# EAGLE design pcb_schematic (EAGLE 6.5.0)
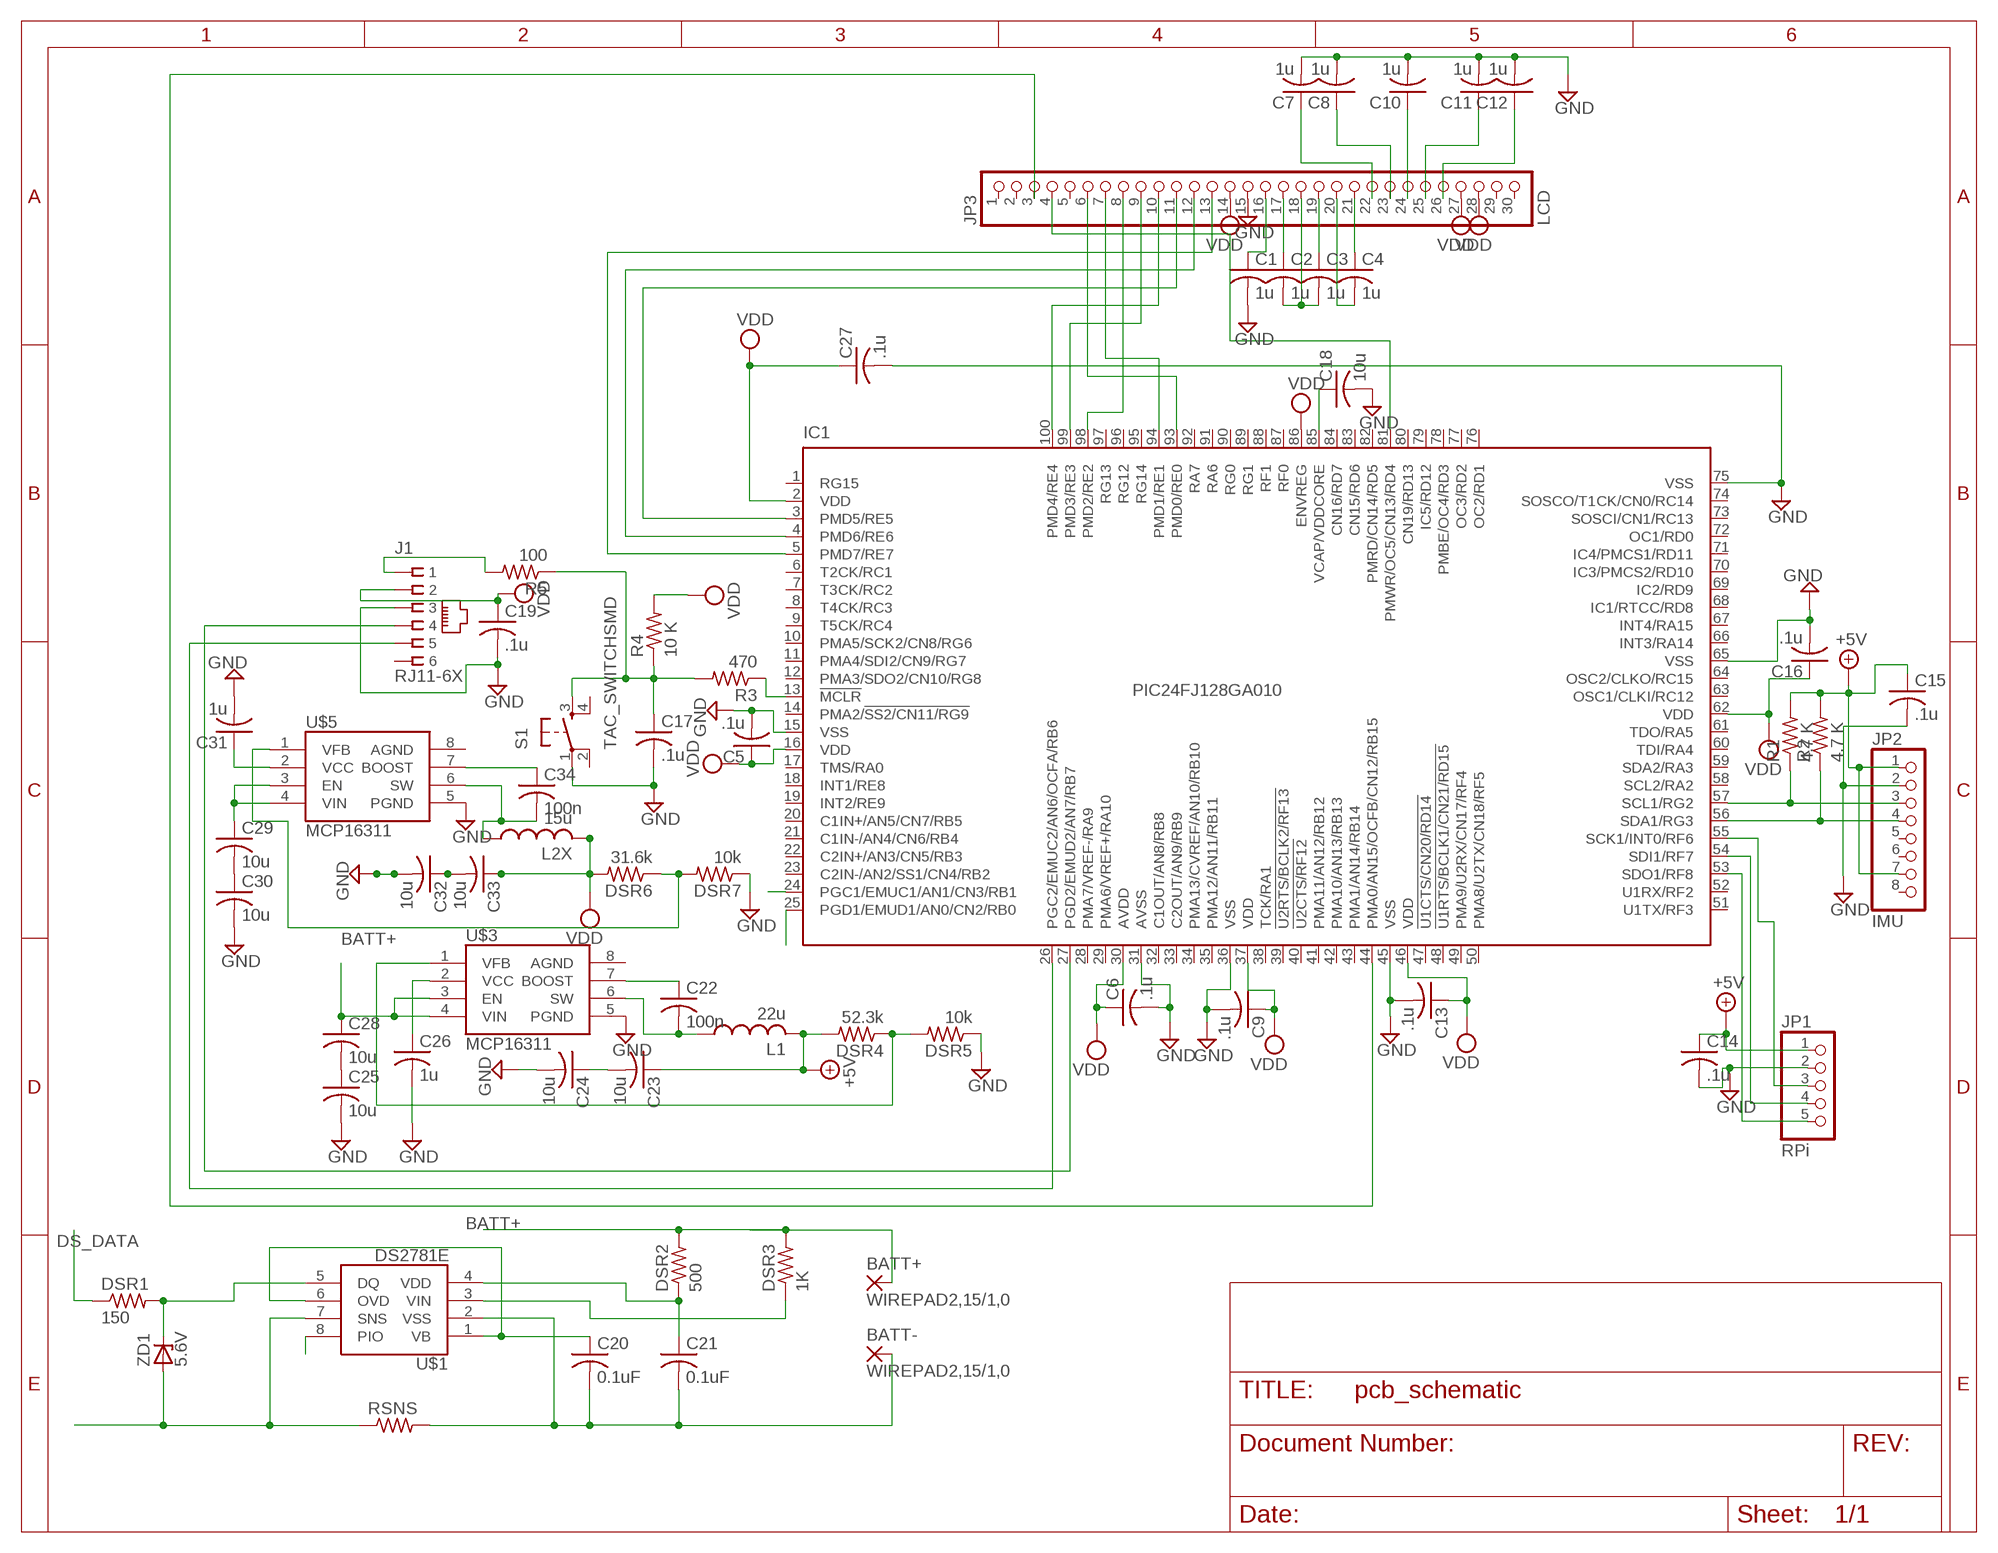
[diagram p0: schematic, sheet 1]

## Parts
BATT+  WIREPAD2,15/1,0  [2,15/1,0]
BATT-  WIREPAD2,15/1,0  [2,15/1,0]
C1  1u  C-USC1206K  [C1206K]
C2  1u  C-USC1206K  [C1206K]
C3  1u  C-USC1206K  [C1206K]
C4  1u  C-USC1206K  [C1206K]
C5  .1u  C-USC1206K  [C1206K]
C6  .1u  C-USC1206K  [C1206K]
C7  1u  C-USC1206K  [C1206K]
C8  1u  C-USC1206K  [C1206K]
C9  .1u  C-USC1206K  [C1206K]
C10  1u  C-USC1206K  [C1206K]
C11  1u  C-USC1206K  [C1206K]
C12  1u  C-USC1206K  [C1206K]
C13  .1u  C-USC1206K  [C1206K]
C14  .1u  C-USC1206K  [C1206K]
C15  .1u  C-USC1206K  [C1206K]
C16  .1u  C-USC1206K  [C1206K]
C17  .1u  C-USC1206K  [C1206K]
C18  10u  C-USC1206K  [C1206K]
C19  .1u  C-USC1206K  [C1206K]
C20  0.1uF  C-US025-024X044  [C025-024X044]
C21  0.1uF  C-US025-024X044  [C025-024X044]
C22  100n  C-US025-024X044  [C025-024X044]
C23  10u  C-US025-024X044  [C025-024X044]
C24  10u  C-US025-024X044  [C025-024X044]
C25  10u  C-US025-024X044  [C025-024X044]
C26  1u  C-US025-024X044  [C025-024X044]
C27  .1u  C-USC1206K  [C1206K]
C28  10u  C-US025-024X044  [C025-024X044]
C29  10u  C-US025-024X044  [C025-024X044]
C30  10u  C-US025-024X044  [C025-024X044]
C31  1u  C-US025-024X044  [C025-024X044]
C32  10u  C-US025-024X044  [C025-024X044]
C33  10u  C-US025-024X044  [C025-024X044]
C34  100n  C-US025-024X044  [C025-024X044]
DSR1  150  R-US_M2012  [M2012]
DSR2  500  R-US_M2012  [M2012]
DSR3  1K  R-US_M2012  [M2012]
DSR4  52.3k  R-US_M2012  [M2012]
DSR5  10k  R-US_M2012  [M2012]
DSR6  31.6k  R-US_M2012  [M2012]
DSR7  10k  R-US_M2012  [M2012]
IC1  PIC24FJ128GA010  [TQFP100-14X14]
J1  RJ11-6X  [RJ11-NO_SHIELD]
JP1  RPi  PINHD-1X5  [1X05]
JP2  IMU  PINHD-1X8  [1X08]
JP3  LCD  PINHD-1X30  [1X30]
L1  22u  L-US0204/5  [0204/5]
L2X  15u  L-US0204/5  [0204/5]
R1  4.7 K  R-US_M2012  [M2012]
R2  4.7 K  R-US_M2012  [M2012]
R3  470  R-US_M2012  [M2012]
R4  10 K  R-US_M2012  [M2012]
R5  100  R-US_M2012  [M2012]
RSNS  R-US_M2012  [M2012]
S1  TAC_SWITCHSMD  [TACTILE-SWITCH-SMD]
U$1  DS2781E  [TSSOP8]
U$3  MCP16311  [MSOP8]
U$5  MCP16311  [MSOP8]
ZD1  5.6V  ZENER-DIODESOD80C  [SOD80C]

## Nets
+5V: C14.1 C15.1 C23.1 DSR4.2 JP1.1 JP2.1 JP2.7 L1.2 R1.2 R2.2
BATT+: BATT+.1(P) C28.1 C29.1 DSR2.2 DSR3.2 U$3.3(EN) U$3.4(VIN) U$5.3(EN) U$5.4(VIN)
DS_DATA: DSR1.1 IC1.25(PGD1/EMUD1/AN0/CN2/RB0)
DS_PACK-: RSNS.1 U$1.7(SNS) ZD1.A
GND: C1.2 C5.2 C6.2 C7.2 C8.2 C9.2 C10.2 C11.2 C12.2 C13.2 C14.2 C15.2 C16.2 C17.2 C18.2 C19.2 C24.2 C25.2 C26.2 C27.2 C30.2 C31.2 C32.2 DSR5.1 DSR7.1 IC1.15(VSS) IC1.31(AVSS) IC1.36(VSS) IC1.45(VSS) IC1.65(VSS) IC1.75(VSS) J1.3 JP1.2 JP2.2 JP3.15 S1.1 U$3.5(PGND) U$5.5(PGND)
N$1: IC1.57(SCL1/RG2) JP2.3 R1.1
N$2: IC1.56(SDA1/RG3) JP2.4 R2.1
N$3: IC1.44(PMA0/AN15/OCFB/CN12/RB15) JP3.3
N$4: IC1.55(SCK1/INT0/RF6) JP1.3
N$5: IC1.54(SDI1/RF7) JP1.4
N$6: IC1.53(SDO1/RF8) JP1.5
N$7: C18.1 IC1.85(VCAP/VDDCORE)
N$8: IC1.5(PMD7/RE7) JP3.13
N$9: IC1.4(PMD6/RE6) JP3.12
N$10: IC1.3(PMD5/RE5) JP3.11
N$11: IC1.100(PMD4/RE4) JP3.10
N$12: IC1.99(PMD3/RE3) JP3.9
N$13: IC1.98(PMD2/RE2) JP3.8
N$14: IC1.94(PMD1/RE1) JP3.7
N$15: IC1.93(PMD0/RE0) JP3.6
N$16: C7.1 JP3.22
N$17: C3.1 JP3.19
N$18: IC1.81(PMWR/OC5/CN13/RD4) JP3.4
N$19: C2.1 JP3.17
N$20: C2.2 C3.2 JP3.18
N$21: C1.1 JP3.16
N$22: C4.2 JP3.20
N$23: C4.1 JP3.21
N$24: C8.1 JP3.23
N$25: C10.1 JP3.24
N$26: C11.1 JP3.25
N$27: C12.1 JP3.26
N$29: J1.1 R5.2
N$30: C25.1 C28.2
N$31: DSR1.2 U$1.5(DQ) ZD1.C
N$32: IC1.26(PGC2/EMUC2/AN6/OCFA/RB6) J1.5
N$33: IC1.27(PGD2/EMUD2/AN7/RB7) J1.4
N$34: C17.1 R3.2 R4.1 R5.1 S1.3
N$35: BATT-.1(P) C20.2 C21.2 RSNS.2 U$1.2(VSS)
N$36: C21.1 DSR2.1 U$1.4(VDD)
N$37: C20.1 U$1.1(VB) U$1.6(OVD)
N$38: C22.2 L1.1 U$3.6(SW)
N$39: DSR3.1 U$1.3(VIN)
N$40: C22.1 U$3.7(BOOST)
N$41: DSR4.1 DSR5.2 U$3.1(VFB)
N$42: C23.2 C24.1
N$43: C26.1 U$3.2(VCC)
N$44: C29.2 C30.1
N$45: C32.1 C33.2
N$46: DSR6.1 DSR7.2 U$5.1(VFB)
N$47: C34.2 L2X.1 U$5.6(SW)
N$48: C34.1 U$5.7(BOOST)
N$49: C31.1 U$5.2(VCC)
N$50: IC1.13(!MCLR) R3.1
PIO: IC1.24(PGC1/EMUC1/AN1/CN3/RB1) U$1.8(PIO)
VDD: C5.1 C6.1 C9.1 C13.1 C16.1 C19.1 C27.1 C33.1 DSR6.2 IC1.2(VDD) IC1.16(VDD) IC1.30(AVDD) IC1.37(VDD) IC1.46(VDD) IC1.62(VDD) IC1.86(ENVREG) J1.2 JP3.14 JP3.27 JP3.28 L2X.2 R4.2
Unconnected: IC1.1(RG15) IC1.6(T2CK/RC1) IC1.7(T3CK/RC2) IC1.8(T4CK/RC3) IC1.9(T5CK/RC4) IC1.10(PMA5/SCK2/CN8/RG6) IC1.11(PMA4/SDI2/CN9/RG7) IC1.12(PMA3/SDO2/CN10/RG8) IC1.14(PMA2/!SS2/CN11/RG9) IC1.17(TMS/RA0) IC1.18(INT1/RE8) IC1.19(INT2/RE9) IC1.20(C1IN+/AN5/CN7/RB5) IC1.21(C1IN-/AN4/CN6/RB4) IC1.22(C2IN+/AN3/CN5/RB3) IC1.23(C2IN-/AN2/SS1/CN4/RB2) IC1.28(PMA7/VREF-/RA9) IC1.29(PMA6/VREF+/RA10) IC1.32(C1OUT/AN8/RB8) IC1.33(C2OUT/AN9/RB9) IC1.34(PMA13/CVREF/AN10/RB10) IC1.35(PMA12/AN11/RB11) IC1.38(TCK/RA1) IC1.39(!U2RTS/BCLK2/RF13) IC1.40(!U2CTS/RF12) IC1.41(PMA11/AN12/RB12) IC1.42(PMA10/AN13/RB13) IC1.43(PMA1/AN14/RB14) IC1.47(!U1CTS/CN20/RD14) IC1.48(!U1RTS/BCLK1/CN21/RD15) IC1.49(PMA9/U2RX/CN17/RF4) IC1.50(PMA8/U2TX/CN18/RF5) IC1.51(U1TX/RF3) IC1.52(U1RX/RF2) IC1.58(SCL2/RA2) IC1.59(SDA2/RA3) IC1.60(TDI/RA4) IC1.61(TDO/RA5) IC1.63(OSC1/CLKI/RC12) IC1.64(OSC2/CLKO/RC15) IC1.66(INT3/RA14) IC1.67(INT4/RA15) IC1.68(IC1/RTCC/RD8) IC1.69(IC2/RD9) IC1.70(IC3/PMCS2/RD10) IC1.71(IC4/PMCS1/RD11) IC1.72(OC1/RD0) IC1.73(SOSCI/CN1/RC13) IC1.74(SOSCO/T1CK/CN0/RC14) IC1.76(OC2/RD1) IC1.77(OC3/RD2) IC1.78(PMBE/OC4/RD3) IC1.79(IC5/RD12) IC1.80(CN19/RD13) IC1.82(PMRD/CN14/RD5) IC1.83(CN15/RD6) IC1.84(CN16/RD7) IC1.87(RF0) IC1.88(RF1) IC1.89(RG1) IC1.90(RG0) IC1.91(RA6) IC1.92(RA7) IC1.95(RG14) IC1.96(RG12) IC1.97(RG13) J1.6 JP2.5 JP2.6 JP2.8 JP3.1 JP3.2 JP3.5 JP3.29 JP3.30 S1.2 S1.4 U$3.8(AGND) U$5.8(AGND)

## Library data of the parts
BATT+ BATT- = wirepad:WIREPAD: Wire PAD connect wire on PCB
C1-C34 = rcl:C-US: CAPACITOR, American symbol
DSR1-DSR7 R1-R5 RSNS = rcl:R-US_: RESISTOR, American symbol
IC1 = microchip:PIC24FJ*GA010: 64/80/100-Pin General Purpose, 16-Bit Flash Microcontrollers Source: http://ww1.microchip.com/downloads/en/DeviceDoc/39747d.pdf; MPN: PIC24FJ128GA010-I/PT; OC_FARNELL: 1146522; OC_NEWARK: 56K7341
J1 = con-tycoelectronics:RJ11: CORCOM Modular RJ Jacks No Shield Source: www.tycoelectronics.com .. ENG_DS_1654001_1099_RJ_L_0507.pdf; MPN: RJ11-6X; OC_FARNELL: unknown; OC_NEWARK: 16R6089
JP1 = pinhead:PINHD-1X5: PIN HEADER
JP2 = pinhead:PINHD-1X8: PIN HEADER
JP3 = pinhead:PINHD-1X30: PIN HEADER
L1 L2X = rcl:L-US: INDUCTOR, American symbol
S1 = SparkFun-Retired:TAC_SWITCH: Momentary Switch Button commonly used for reset or general input. Spark Fun Electronics SKU : COM-00097 SMT- SWCH-08247; PROD_ID: SWCH-08247
U$1 = fuelgauge:DS2781E
U$3 U$5 = fuelgauge:MCP16311
ZD1 = diode:ZENER-DIODE: Z-Diode

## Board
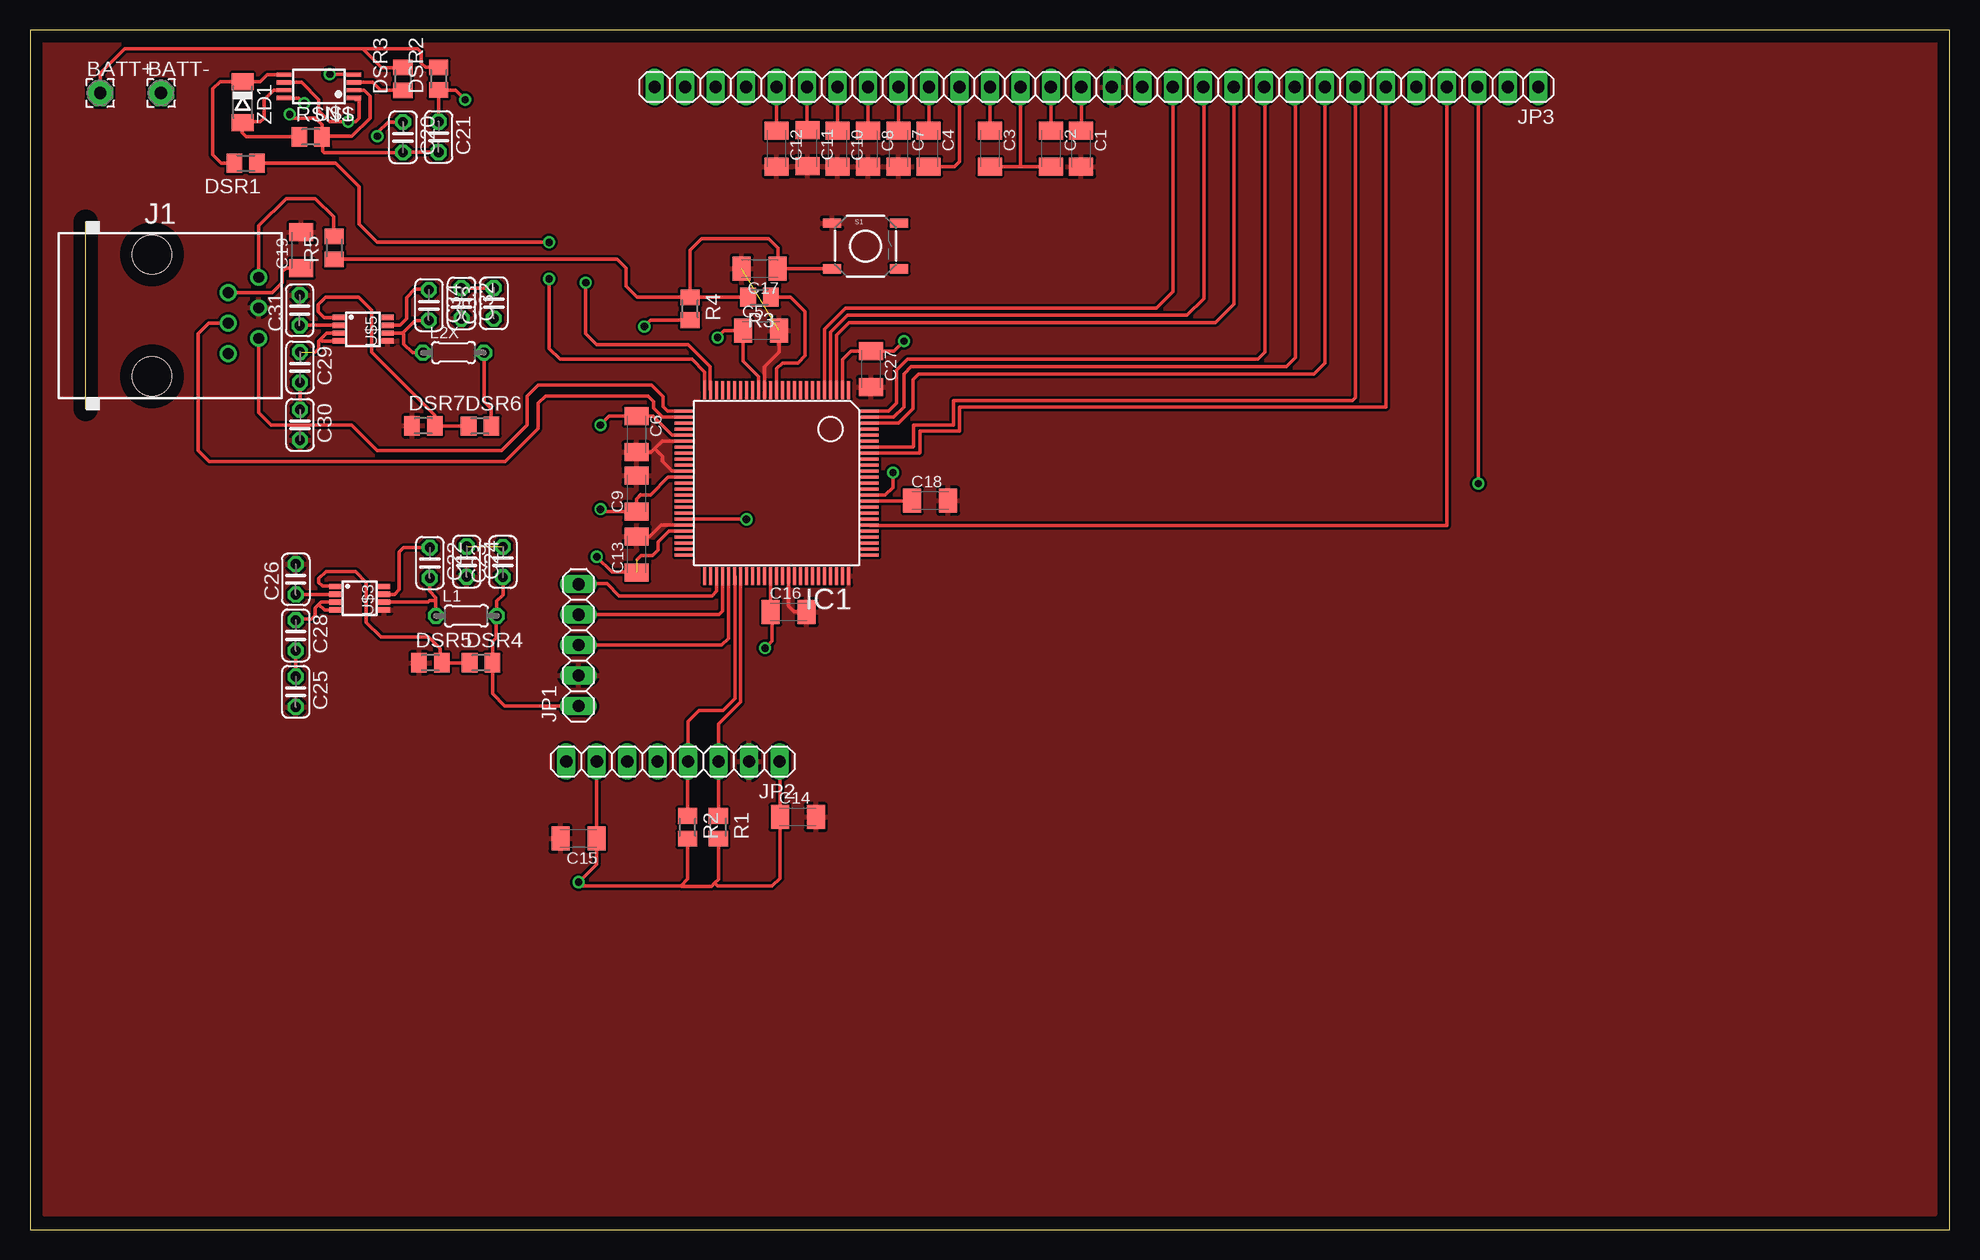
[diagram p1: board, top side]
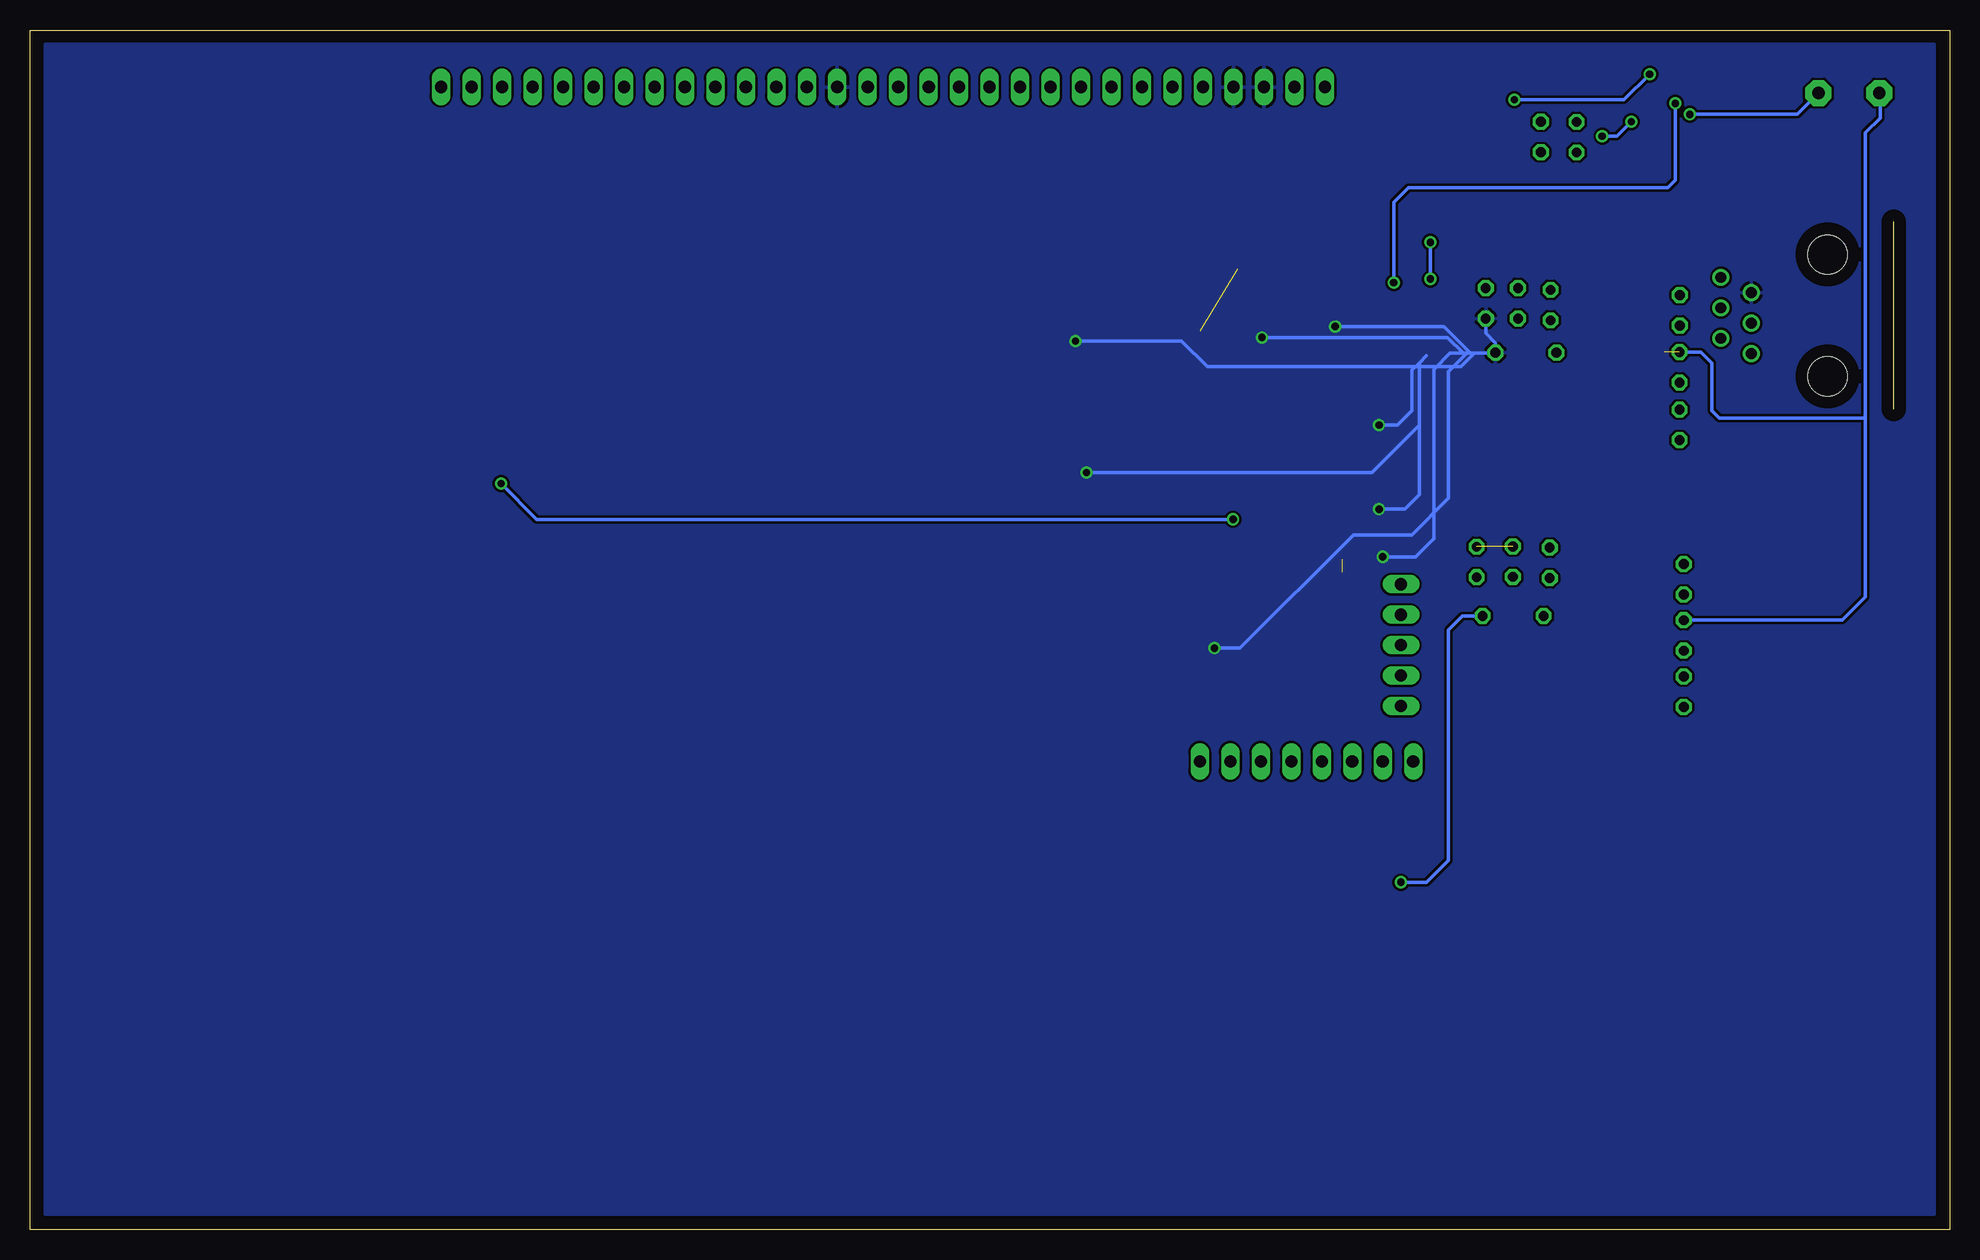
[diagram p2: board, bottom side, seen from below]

Size 160 x 100 mm. Coordinates in mm from the lower left corner, seen from the top.
Outline: 0,0 160,0 160,100 0,100 0,0
Copper layers (1*16): Top 0.035mm / dielectric 1.5mm / Bottom 0.035mm
Design rules "default": minimum track width 10mil, minimum drill 24mil, track to track 8mil, track to pad 8mil, pad to pad 8mil, via to via 8mil, smd to smd 8mil, copper to edge 40mil, drill to drill 8mil, minimum pad ring 10mil, minimum via ring 8mil, stop-mask expansion 4mil, vias tented up to drill 0mil, thermal gap 10mil

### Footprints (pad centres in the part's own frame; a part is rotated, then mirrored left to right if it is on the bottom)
2,15/1,0 = drill 1.016 pad 2.159 octagon: 1 0,0
C1206K = smd 1.5 x 2: 1 -1.5,0; 2 1.5,0
C025-024X044 = drill 0.813 octagon: 1 -1.27,0; 2 1.27,0
M2012 = smd 1.3 x 1.6: 1 -0.95,0; 2 0.95,0
TQFP100-14X14 = smd 0.27 x 1.5: 1 -6,-7.75; 2 -5.5,-7.75; 3 -5,-7.75; 4 -4.5,-7.75; 5 -4,-7.75; 6 -3.5,-7.75; 7 -3,-7.75; 8 -2.5,-7.75; 9 -2,-7.75; 10 -1.5,-7.75; 11 -1,-7.75; 12 -0.5,-7.75; 13 0,-7.75; 14 0.5,-7.75; 15 1,-7.75; 16 1.5,-7.75; 17 2,-7.75; 18 2.5,-7.75; 19 3,-7.75; 20 3.5,-7.75; 21 4,-7.75; 22 4.5,-7.75; 23 5,-7.75; 24 5.5,-7.75; 25 6,-7.75; 51 6,7.75; 52 5.5,7.75; 53 5,7.75; 54 4.5,7.75; 55 4,7.75; 56 3.5,7.75; 57 3,7.75; 58 2.5,7.75; 59 2,7.75; 60 1.5,7.75; 61 1,7.75; 62 0.5,7.75; 63 0,7.75; 64 -0.5,7.75; 65 -1,7.75; 66 -1.5,7.75; 67 -2,7.75; 68 -2.5,7.75; 69 -3,7.75; 70 -3.5,7.75; 71 -4,7.75; 72 -4.5,7.75; 73 -5,7.75; 74 -5.5,7.75; 75 -6,7.75 | smd 1.5 x 0.27: 26 7.75,-6; 27 7.75,-5.5; 28 7.75,-5; 29 7.75,-4.5; 30 7.75,-4; 31 7.75,-3.5; 32 7.75,-3; 33 7.75,-2.5; 34 7.75,-2; 35 7.75,-1.5; 36 7.75,-1; 37 7.75,-0.5; 38 7.75,0; 39 7.75,0.5; 40 7.75,1; 41 7.75,1.5; 42 7.75,2; 43 7.75,2.5; 44 7.75,3; 45 7.75,3.5; 46 7.75,4; 47 7.75,4.5; 48 7.75,5; 49 7.75,5.5; 50 7.75,6; 76 -7.75,6; 77 -7.75,5.5; 78 -7.75,5; 79 -7.75,4.5; 80 -7.75,4; 81 -7.75,3.5; 82 -7.75,3; 83 -7.75,2.5; 84 -7.75,2; 85 -7.75,1.5; 86 -7.75,1; 87 -7.75,0.5; 88 -7.75,0; 89 -7.75,-0.5; 90 -7.75,-1; 91 -7.75,-1.5; 92 -7.75,-2; 93 -7.75,-2.5; 94 -7.75,-3; 95 -7.75,-3.5; 96 -7.75,-4; 97 -7.75,-4.5; 98 -7.75,-5; 99 -7.75,-5.5; 100 -7.75,-6
RJ11-NO_SHIELD = drill 0.9 pad 1.4: 1 -3.175,8.89; 2 -1.905,6.35; 3 -0.635,8.89; 4 0.635,6.35; 5 1.905,8.89; 6 3.175,6.35 | hole 3.251: -5.08,0; 5.08,0
1X05 = drill 1.016 long: 1 -5.08,0; 2 -2.54,0; 3 0,0; 4 2.54,0; 5 5.08,0
1X08 = drill 1.016 long: 1 -8.89,0; 2 -6.35,0; 3 -3.81,0; 4 -1.27,0; 5 1.27,0; 6 3.81,0; 7 6.35,0; 8 8.89,0
1X30 = drill 1.016 long: 1 -36.83,0; 2 -34.29,0; 3 -31.75,0; 4 -29.21,0; 5 -26.67,0; 6 -24.13,0; 7 -21.59,0; 8 -19.05,0; 9 -16.51,0; 10 -13.97,0; 11 -11.43,0; 12 -8.89,0; 13 -6.35,0; 14 -3.81,0; 15 -1.27,0; 16 1.27,0; 17 3.81,0; 18 6.35,0; 19 8.89,0; 20 11.43,0; 21 13.97,0; 22 16.51,0; 23 19.05,0; 24 21.59,0; 25 24.13,0; 26 26.67,0; 27 29.21,0; 28 31.75,0; 29 34.29,0; 30 36.83,0
0204/5 = drill 0.813 octagon: 1 -2.54,0; 2 2.54,0
TACTILE-SWITCH-SMD = smd 1.524 x 0.762: 1 -2.794,1.905; 2 2.794,1.905; 3 -2.794,-1.905; 4 2.794,-1.905
TSSOP8 = smd 1.2 x 0.35: 1 -2.925,0.975; 2 -2.925,0.325; 3 -2.925,-0.325; 4 -2.925,-0.975; 5 2.925,-0.975; 6 2.925,-0.325; 7 2.925,0.325; 8 2.925,0.975
MSOP8 = smd 0.45 x 1: 1 -0.975,-2.05; 2 -0.325,-2.05; 3 0.325,-2.05; 4 0.975,-2.05; 5 0.975,2.05; 6 0.325,2.05; 7 -0.325,2.05; 8 -0.975,2.05
SOD80C = smd 1.4 x 1.8: A 1.7,0; C -1.7,0

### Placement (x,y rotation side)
BATT+  5.84,94.74 0 top
BATT-  10.92,94.74 0 top
C1  87.6,90.09 270 top
C2  85.09,90.12 270 top
C3  80.01,90.12 270 top
C4  74.9,90.12 270 top
C5  60.93,74.93 0 top
C6  50.55,66.29 270 top
C7  72.39,90.12 270 top
C8  69.85,90.09 270 top
C9  50.55,61.37 90 top
C10  67.31,90.12 270 top
C11  64.82,90.14 270 top
C12  62.23,90.12 270 top
C13  50.57,56.29 90 top
C14  64.01,34.39 0 top
C15  45.72,32.59 180 top
C16  63.25,51.46 0 top
C17  60.83,80.11 180 top
C18  75.03,60.76 0 top
C19  22.61,81.64 90 top
C20  31.09,91.06 270 top
C21  34.06,91.08 270 top
C22  33.32,55.58 270 top
C23  39.42,55.65 90 top
C24  36.4,55.68 270 top
C25  22.15,44.83 270 top
C26  22.15,54.2 90 top
C27  70.1,71.73 270 top
C28  22.15,49.53 270 top
C29  22.5,71.88 270 top
C30  22.5,67.08 270 top
C31  22.48,76.63 90 top
C32  35.97,77.22 270 top
C33  38.66,77.22 90 top
C34  33.25,77.06 270 top
DSR1  17.98,88.9 180 top
DSR2  34.06,95.94 90 top
DSR3  31.09,95.91 90 top
DSR4  37.59,47.24 0 top
DSR5  33.38,47.24 0 top
DSR6  37.52,66.98 0 top
DSR7  32.79,67.01 0 top
IC1  62.23,62.23 180 top
J1  10.16,76.2 270 top
JP1  45.72,48.72 90 top
JP2  53.59,39.01 180 top
JP3  88.9,95.25 180 top
L1  36.37,51.16 0 top
L2X  35.31,73.1 0 top
R1  57.38,33.53 270 top
R2  54.81,33.53 270 top
R3  60.81,77.72 180 top
R4  55.02,76.76 270 top
R5  25.35,81.84 90 top
RSNS  23.39,91.08 0 top
S1  69.65,81.99 0 top
U$1  24.08,95.3 180 top
U$3  27.48,52.63 270 top
U$5  27.76,75.06 270 top
ZD1  17.73,93.98 270 top

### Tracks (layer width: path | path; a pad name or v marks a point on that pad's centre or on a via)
+5V  (via drill 0.6)
  Top 0.305: C23.1 39.42,52.91 38.91,52.4 L1.2 38.86,51.1 38.86,49.33 38.54,49.01 DSR4.2 38.54,44.67 39.55,43.66 45.7,43.66 JP1.1 | JP2.1 62.51,38.99 C14.1 62.51,29.29 61.87,28.65 57.3,28.65 57.07,28.88 | R2.2 54.81,29.21 54.25,28.65 | 54.25,28.65 46.02,28.65 v45.72,28.96 47.22,30.46 C15.1 47.24,32.61 JP2.7 | R1.2 57.38,29.18 57.07,28.88 | 57.07,28.88 56.79,28.6 54.3,28.6 54.25,28.65
  Bottom 0.305: v45.72,28.96 43.59,28.96 41.76,30.79 41.76,49.99 40.59,51.16 L1.2
BATT+  (1 unrouted)
  Top 0.305: U$3.3 24.26,52.3 24.08,52.12 | 24.08,52.12 23.77,51.82 23.77,51.21 23.47,50.9 22.25,50.9 C28.1 | U$3.4 24.55,51.65 24.08,52.12 | DSR3.2 29.33,96.86 27.74,98.45 | 27.74,98.45 7.9,98.45 5.84,96.39 BATT+.1 | DSR2.2 32.96,96.89 32.61,97.23 32.61,98.15 32.31,98.45 27.74,98.45 | U$5.3 24.75,74.73 24.23,74.22 | 24.23,74.22 24.08,74.07 24.08,73.46 23.77,73.15 | U$5.4 24.37,74.08 24.23,74.22
  Bottom 0.305: C28.1 8.94,50.8 7.01,52.73 7.01,67.67 | 7.01,67.67 7.01,91.44 5.79,92.66 5.79,94.69 BATT+.1 | C29.1 20.73,73.15 19.81,72.24 19.81,68.28 19.2,67.67 7.01,67.67
DS_DATA  (via drill 0.6)
  Top 0.305: IC1.25 56.23,71.48 55.17,72.54 44.2,72.54 43.28,73.46 v43.28,79.25 | v43.28,82.3 28.96,82.3 27.43,83.82 27.43,86.94 25.48,88.9 DSR1.1
  Bottom 0.305: v43.28,79.25 v43.28,82.3
DS_PACK-
  Top 0.305: U$1.7 20.3,94.98 19.51,94.18 19.51,92.66 19.2,92.35 17.8,92.35 ZD1.A 17.68,92.23 17.68,91.44 18.03,91.08 RSNS.1
GND  (1 unrouted)
  Top 0.305: IC1.31 52.73,65.73 52.08,65.09 | 52.08,65.09 51.79,64.8 C6.2 | IC1.45 52.61,58.73 51.66,57.78 C13.2 | IC1.65 63.23,51.98 63.7,51.51 64.69,51.51 C16.2 | IC1.15 61.23,71.95 62.43,73.15 C5.2 | IC1.36 53.51,63.23 52.73,64.01 52.73,64.44 52.08,65.09
  pour Top: 1.27,99.06 158.75,99.06 158.75,1.27 1.27,1.27
N$1
  Top 0.305: R1.1 57.38,38.99 JP2.3 57.4,42.16 59.23,43.99 IC1.57
N$2
  Top 0.305: R2.1 54.81,38.96 JP2.4 54.86,42.37 55.78,43.28 57.76,43.28 58.75,44.27 58.75,54.46 IC1.56
N$3  (via drill 0.6)
  Top 0.305: IC1.44 59.69,59.23 v59.72,59.21 | v120.73,62.18 120.73,95.17 JP3.3
  Bottom 0.305: v59.72,59.21 117.75,59.21 v120.73,62.18
N$4
  Top 0.305: IC1.55 58.23,49.29 57.66,48.72 JP1.3
N$5
  Top 0.305: IC1.54 57.73,51.56 57.43,51.26 JP1.4
N$6
  Top 0.305: IC1.53 57.23,53.22 56.84,52.83 49.12,52.83 48.11,53.85 45.77,53.85 JP1.5
N$7
  Top 0.305: IC1.85 73.5,60.73 C18.1
N$8
  Top 0.305: IC1.5 66.23,75.07 67.97,76.81 93.88,76.81 95.28,78.21 95.28,95.22 JP3.13
N$9
  Top 0.305: IC1.4 66.73,74.81 68.15,76.22 96.44,76.22 97.84,77.62 97.84,95.2 JP3.12
N$10
  Top 0.305: IC1.3 67.23,74.55 68.28,75.59 98.81,75.59 100.36,77.14 100.36,95.22 JP3.11
N$11
  Top 0.305: IC1.100 71.58,68.23 72.24,68.89 72.24,71.63 73.15,72.54 102.36,72.54 102.95,73.13 102.95,95.17 JP3.10
N$12
  Top 0.305: IC1.99 72,67.73 72.85,68.58 72.85,71.32 73.46,71.93 104.72,71.93 105.49,72.69 105.49,95.17 JP3.9
N$13
  Top 0.305: IC1.98 72.39,67.23 73.58,68.43 73.58,70.84 74.07,71.32 107.04,71.32 107.92,72.21 107.92,95.22 JP3.8
N$14
  Top 0.305: IC1.94 73.61,65.23 73.66,65.28 73.66,67.06 76.96,67.06 76.96,69.09 110.24,69.09 110.49,69.34 JP3.7
N$15
  Top 0.305: IC1.93 74.13,64.73 74.17,64.77 74.17,66.55 77.47,66.55 77.47,68.58 113.03,68.58 JP3.6
N$16
  Top 0.305: JP3.22 C7.1
N$17
  Top 0.305: JP3.19 C3.1
N$18
  Top 0.305: JP3.4 118.11,58.67 70.04,58.67 IC1.81
N$19
  Top 0.305: C2.1 JP3.17
N$20
  Top 0.305: C3.2 82.6,88.62 | 82.6,88.62 C2.2 | JP3.18 82.55,88.67 82.6,88.62
N$21
  Top 0.305: JP3.16 87.63,91.62 C1.1
N$22
  Top 0.305: JP3.20 77.47,89.03 77.06,88.62 C4.2
N$23
  Top 0.305: JP3.21 74.93,91.64 C4.1
N$24
  Top 0.305: JP3.23 C8.1
N$25
  Top 0.305: JP3.24 C10.1
N$26
  Top 0.305: JP3.25 64.77,91.69 C11.1
N$27
  Top 0.305: JP3.26 C12.1
N$29
  Top 0.305: J1.1 19.05,83.67 21.34,85.95 23.77,85.95 25.3,84.43 25.3,82.84 R5.2
N$30
  Top 0.305: C28.2 C25.1
N$31
  Top 0.305: U$1.5 19.77,96.28 19.2,95.71 17.76,95.71 ZD1.C 17.7,95.71 15.85,95.71 15.24,95.1 15.24,89.61 15.95,88.9 DSR1.2
N$32
  Top 0.305: J1.5 19.05,68.12 20.12,67.06 26.82,67.06 28.96,64.92 39.32,64.92 41.45,67.06 41.45,69.49 42.37,70.41 51.82,70.41 52.78,69.44 52.78,68.61 53.16,68.23 IC1.26
N$33
  Top 0.305: J1.4 14.91,75.56 14.02,74.68 14.02,64.92 14.94,64.01 39.62,64.01 42.37,66.75 42.37,68.89 42.98,69.49 51.54,69.49 51.99,69.04 51.99,68.48 52.73,67.74 54.47,67.74 IC1.27
N$34
  Top 0.305: S1.3 62.36,80.09 | 62.36,80.09 C17.1 | R3.2 55.03,77.72 R4.1 | 62.36,80.09 62.36,81.81 61.57,82.6 55.98,82.6 55.02,81.64 R4.1 | R5.1 48.96,80.89 49.68,80.16 49.68,78.64 50.6,77.72 55,77.72 R4.1
N$35  (via drill 0.6)
  Top 0.305: U$1.2 27.86,94.98 28.35,94.49 28.35,92.66 26.82,91.14 24.39,91.14 RSNS.2 | RSNS.2 24.38,91.04 24.38,89.92 24.51,89.79 C20.2 31.11,89.81 C21.2 | RSNS.2 24.34,92.09 23.77,92.66 21.95,92.66 v21.64,92.96
  Bottom 0.305: v21.64,92.96 12.7,92.96 BATT-.1
N$36  (via drill 0.6)
  Top 0.305: C21.1 DSR2.1 35.47,94.99 v36.27,94.18 | v24.99,96.32 26.96,96.32 U$1.4
  Bottom 0.305: v36.27,94.18 27.13,94.18 v24.99,96.32
N$37  (via drill 0.6)
  Top 0.305: C20.1 29.84,92.33 28.96,91.44 v28.96,91.14 | U$1.1 27.15,94.18 27.43,94.18 27.43,92.66 27.13,92.35 v26.52,92.35 24.99,92.35 24.08,93.27 24.08,94.18 22.64,95.63 U$1.6
  Bottom 0.305: v28.96,91.14 27.74,91.14 v26.52,92.35
N$38
  Top 0.305: U$3.6 33.2,52.3 33.33,52.43 33.83,52.43 | C22.2 33.33,53.21 33.83,52.7 33.83,52.43 | 33.83,52.43 L1.1
N$39
  Top 0.305: U$1.3 28.55,95.63 29.21,94.97 31.08,94.97 DSR3.1
N$40
  Top 0.305: U$3.7 30.4,52.95 30.79,53.34 30.79,56.46 31.17,56.84 C22.1
N$41
  Top 0.305: U$3.1 25.39,53.65 24.38,53.65 24.08,53.95 24.08,54.25 24.69,54.86 27.13,54.86 28.04,53.95 28.04,50.6 29.26,49.38 33.22,49.38 34.17,48.43 34.17,47.4 DSR5.2 DSR4.1
N$42  (1 unrouted)
N$43
  Top 0.305: U$3.2 22.17,52.95 C26.1
N$44
  Top 0.305: C29.2 22.53,69.32 C30.1
N$45
  Top 0.305: C33.2 C32.1
N$46
  Top 0.305: DSR6.1 33.77,66.98 DSR7.2 33.74,67.88 28.5,73.13 28.5,76.63 27.41,77.72 24.64,77.72 24.03,77.11 24.03,76.5 24.51,76.02 U$5.1
N$47
  Top 0.305: U$5.6 31.07,74.73 | 31.07,74.73 32.11,75.77 33.22,75.77 C34.2 | L2X.1 31.88,73.1 31.17,73.81 31.17,74.64 31.07,74.73
N$48
  Top 0.305: U$5.7 30.86,75.38 31.39,75.92 31.39,77.7 32.08,78.38 33.2,78.38 C34.1
N$49
  Top 0.305: U$5.2 22.31,75.38 C31.1
N$50
  Top 0.305: R3.1 63.4,77.72 64.62,76.5 64.62,72.85 64.01,72.24 62.71,72.24 62.23,71.75 IC1.13
PIO  (via drill 0.6)
  Top 0.305: U$1.8 22.41,94.33 v22.86,93.88 | v46.33,78.94 46.33,74.68 47.24,73.76 54.86,73.76 56.69,71.93 56.69,70.02 IC1.24
  Bottom 0.305: v22.86,93.88 22.86,87.48 23.47,86.87 45.11,86.87 46.33,85.65 v46.33,78.94
VDD  (via drill 0.6)  (1 unrouted)
  Top 0.305: IC1.16 60.73,71.1 59.44,72.39 59.44,74.91 C5.1 57.86,74.93 v57.3,74.37 | IC1.37 53.2,62.73 51.71,61.24 50.9,61.24 50.55,60.88 C9.1 | J1.2 20.19,78.11 21.03,78.94 21.03,79.86 21.34,80.16 22.58,80.16 C19.1 | IC1.30 53.51,66.23 51.94,67.79 C6.1 | C6.1 | IC1.46 53.25,58.23 52.35,57.33 52.35,56.64 51.89,56.19 50.93,56.19 50.6,55.85 | C13.1 50.6,54.81 48.52,54.81 v47.24,56.08 | C9.1 50.55,60.91 50.9,61.27 | C16.1 61.73,51.48 IC1.62 61.73,51.35 61.87,51.21 61.87,49.07 v61.27,48.46 | IC1.2 67.73,72.5 68.45,73.23 C27.1 72.01,73.23 v72.85,74.07 | L2X.2 37.85,69.04 38.46,68.43 38.46,66.99 DSR6.2 | C6.1 48.28,67.79 v47.55,67.06 | C9.1 47.73,59.87 v47.55,60.05 | R4.2 51.73,75.81 v51.21,75.29 | IC1.86 71.29,61.23 71.93,61.87 v71.93,63.09
  Bottom 0.305: C33.1 38.66,74.73 37.85,73.91 L2X.2 37.9,73.05 39.62,73.05 | v47.55,67.06 46.02,67.06 44.81,68.28 44.81,71.63 44.2,72.24 | v47.55,60.05 45.41,60.05 44.2,61.27 44.2,67.06 | 44.2,67.06 44.2,72.24 | 44.2,72.24 43.59,72.85 | v47.24,56.08 44.5,56.08 42.98,57.61 42.98,71.7 41.63,73.05 40.54,73.05 | 40.54,73.05 40.23,73.05 | 40.23,73.05 39.93,73.05 | 39.93,73.05 39.62,73.05 | v61.27,48.46 59.13,48.46 49.68,57.91 44.81,57.91 41.76,60.96 41.76,71.53 40.23,73.05 | v57.3,74.37 41.86,74.37 40.54,73.05 | v51.21,75.29 42.16,75.29 39.93,73.05 | v72.85,74.07 64.01,74.07 61.87,71.93 40.74,71.93 39.62,73.05 | v71.93,63.09 48.16,63.09 44.2,67.06
  pour Bottom: 1.27,98.81 158.75,98.81 158.75,95.25 158.75,1.27 142.24,1.27 1.27,1.27 1.27,2.54 1.27,25.65

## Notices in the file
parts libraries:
SparkFun-Retired: Licensing:Creative Commons ShareAlike 4.0 International - https://creativecommons.org/licenses/by-sa/4.0
